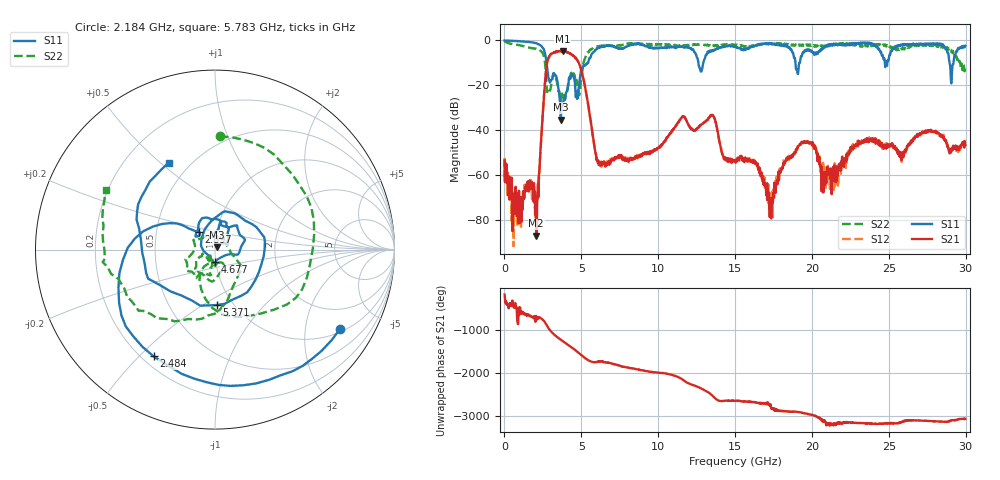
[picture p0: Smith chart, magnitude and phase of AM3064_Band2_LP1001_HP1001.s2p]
# Hz S DB R 50.0
!freq dBS11 angS11 dBS21 angS21 dBS12 angS12 dBS22 angS22
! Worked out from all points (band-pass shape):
!   1600 points, 10 MHz to 29.98 GHz, reference 50 ohm
!   highest |S21| = -4.70 dB at 3.777 GHz (marker M1); lowest = -86.8 dB at 2.072 GHz (marker M2)
!   |S21| within 3 dB of the highest: 2.868 GHz to 4.624 GHz (1.756 GHz wide, 46.9 % of centre)
!   lowest |S11| = -35.1 dB at 3.665 GHz (marker M3), VSWR 1.04, Z = 51.3 + j1.22 ohm
!   |S11| at or under -10 dB: 2.733 GHz to 5.395 GHz (2.662 GHz wide, 65.5 % of centre); 12.61 GHz to 12.93 GHz (318.6 MHz wide, 2.49 % of centre); 28.95 GHz to 29.2 GHz (253 MHz wide, 0.87 % of centre)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
!   |S22| runs from -27.5 to -0.2 dB; largest |S21 - S12| = 0.02
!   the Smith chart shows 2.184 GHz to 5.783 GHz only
!   S11 on the Smith chart (normalised r, x): 2.184 GHz: 1.10, -3.05; 2.484 GHz: 0.25, -0.55; 2.897 GHz: 0.82, +0.17; 4.677 GHz: 0.99, -0.14; 5.371 GHz: 0.84, -0.57; 5.783 GHz: 0.38, +0.53
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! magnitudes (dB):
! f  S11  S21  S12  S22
! 10 MHz  0.0  -53.3  -52.3  -0.2
! 572.3 MHz  -0.2  -70.0  -74.4  -1.7
! 2.072 GHz  -1.3  -86.8  -67.7  -3.7
! 2.184 GHz  -1.7  -63.9  -61.9  -4.0
! 2.484 GHz  -3.3  -33.3  -33.3  -5.5
! 2.897 GHz  -17.4  -7.3  -7.2  -21.2
! 3.665 GHz  -35.1  -4.7  -4.8  -26.1
! 3.777 GHz  -28.8  -4.7  -4.9  -25.3
! 4.677 GHz  -23.1  -8.2  -8.2  -17.6
! 5.015 GHz  -13.0  -13.7  -13.7  -14.9
! 5.371 GHz  -10.2  -25.5  -25.5  -5.9
! 5.783 GHz  -5.2  -44.0  -43.9  -3.2
! 6.252 GHz  -2.9  -55.7  -53.9  -2.4
! 10 GHz  -3.4  -47.7  -47.7  -1.8
! 13.51 GHz  -4.4  -33.1  -33.2  -2.5
! 15 GHz  -2.7  -53.6  -53.5  -1.8
! 16.32 GHz  -2.2  -54.8  -54.1  -2.2
! 17.37 GHz  -1.6  -73.6  -74.2  -1.2
! 19.99 GHz  -4.8  -45.8  -46.0  -1.9
! 21.25 GHz  -1.7  -57.7  -65.1  -2.3
! 25 GHz  -8.6  -46.7  -46.5  -2.3
! 29.98 GHz  -2.4  -46.3  -46.1  -10.9
